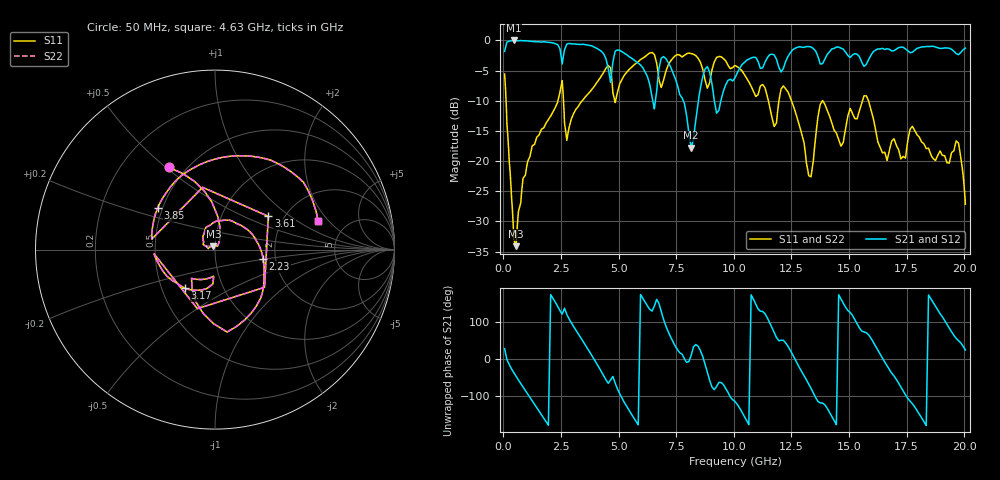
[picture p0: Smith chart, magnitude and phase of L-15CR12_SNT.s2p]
#	mhz	s	ma	r	50
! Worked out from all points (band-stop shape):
!   1001 points, 50 MHz to 20.05 GHz, reference 50 ohm
!   highest |S21| = -0.01 dB at 450 MHz (marker M1); lowest = -17.8 dB at 8.15 GHz (marker M2)
!   |S21| within 3 dB of the highest: start of sweep to 2.518 GHz; 15.87 GHz to end of sweep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
!   lowest |S11| = -34.1 dB at 550 MHz (marker M3), VSWR 1.04, Z = 49.1 + j1.73 ohm
!   |S11| at or under -10 dB: 114.5 MHz to 2.364 GHz (2.249 GHz wide, 182 % of centre); 13.86 GHz to 15.58 GHz (1.724 GHz wide, 11.7 % of centre); 15.84 GHz to end of sweep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
!   |S22| runs from -34.1 to -2.0 dB; largest |S21 - S12| = 0
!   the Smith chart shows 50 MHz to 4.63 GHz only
!   S11 on the Smith chart (normalised r, x): 50 MHz: 0.40, +0.51; 2.23 GHz: 1.72, -0.19; 3.17 GHz: 0.66, -0.30; 3.61 GHz: 1.66, +0.70; 3.85 GHz: 0.47, +0.26; 4.63 GHz: 3.11, +1.56
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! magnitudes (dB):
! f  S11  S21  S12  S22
! 50 MHz  -5.6  -1.8  -1.8  -5.6
! 450 MHz  -33.0  0.0  0.0  -33.0
! 550 MHz  -34.1  -0.1  -0.1  -34.1
! 2.23 GHz  -11.3  -0.5  -0.5  -11.3
! 3.17 GHz  -11.3  -0.6  -0.6  -11.3
! 3.39 GHz  -10.1  -0.7  -0.7  -10.1
! 3.61 GHz  -9.1  -0.8  -0.8  -9.1
! 3.85 GHz  -8.1  -0.9  -0.9  -8.1
! 4.63 GHz  -4.5  -6.5  -6.5  -4.5
! 6.73 GHz  -5.9  -5.3  -5.3  -5.9
! 8.15 GHz  -2.2  -17.8  -17.8  -2.2
! 8.77 GHz  -6.8  -4.7  -4.7  -6.8
! 10.05 GHz  -4.2  -6.2  -6.2  -4.2
! 11.75 GHz  -14.3  -2.4  -2.4  -14.3
! 12.25 GHz  -8.1  -3.5  -3.5  -8.1
! 13.39 GHz  -21.5  -1.2  -1.2  -21.5
! 13.85 GHz  -10.0  -3.9  -3.9  -10.0
! 14.67 GHz  -17.4  -1.3  -1.3  -17.4
! 15.73 GHz  -9.2  -4.0  -4.0  -9.2
! 16.73 GHz  -18.6  -1.4  -1.4  -18.6
! 19.69 GHz  -16.8  -2.3  -2.3  -16.8
! 20.05 GHz  -27.2  -1.3  -1.3  -27.2
